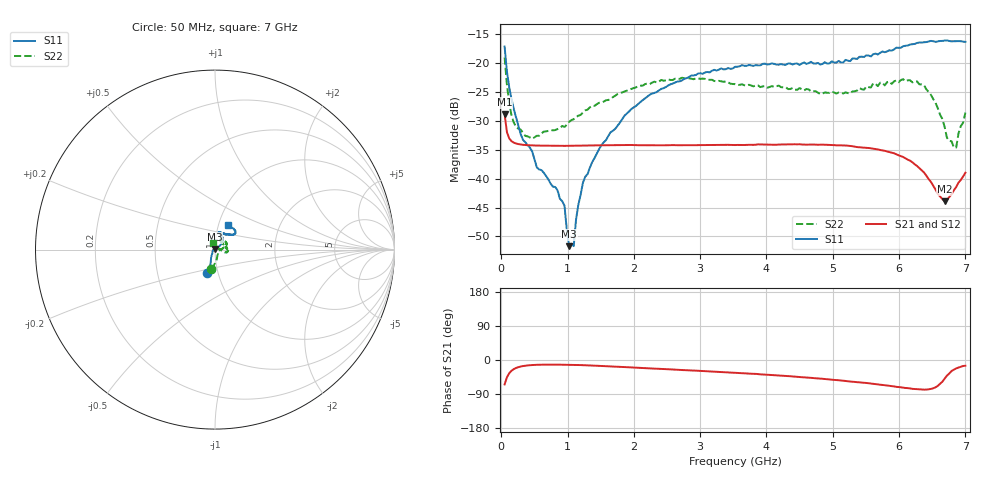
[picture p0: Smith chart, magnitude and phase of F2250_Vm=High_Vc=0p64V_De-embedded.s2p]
! Integrated Device Technology
! Corporate Headquarters
! 6024 Silver Creek Valley Road
! San Jose, CA 95138  USA
! Phone:  1-408-284-8200
! Toll Free:  1-800-223-1366
! Webpage:  http://www.idt.com/
! Timing and RF Division
! 515 Groton Road, Suite 102
! Westford, MA 01886-6024
! Device:  F2250
! Description: Voltage Variable RF Attenuator
! Frequency:  50.0 -  6000.00 MHz
! Package:  3x3 mm Thin QFN Plastic Package: 16 pin
! Ports:  2 RF, 3 DC
!  Pin  1  = GND
!  Pin  2  = NC
!  Pin  3  = RF1  = Port 1
!  Pin  4  = NC
!  Pin  5  = GND
!  Pin  6  = GND
!  Pin  7  = GND
!  Pin  8  = GND
!  Pin  9  = NC
!  Pin 10  = RF2  = Port 2
!  Pin 11  = NC
!  Pin 12  = GND
!  Pin 13  = GND
!  Pin 14  = VCNTRL
!  Pin 15  = VDD
!  Pin 16  = VMODE
! Vcntrl:  0.640 Volts
! Vmode:  +3.300 Volts
! Vdd:  +3.30  Volts
! Current:  1.281 mA
! Data:  The device was measured on a the F2250 evaluation board which has
!  individual transmission lines to the RF pins.  Data was collected
!  using a calibrated network analyzer.  The evaluation board was
!  de-embedded using a TRL calibration technique.
!  The reference plane is the edge of the package pin.
! Misc:  SN 10
!  Action Tracker AT0258
! Date Measured:  2014-11-26
! Date:  2015-10-15  MJV
! Note:
!  Integrated Device Technology supplies this data as a sample of measured
!  data at the package pin for this product.  Your particular data for this
!  product may vary.
!  Data was taken at 25 degrees C.
!  Integrated Device Technology reserves the right to change this data at anytime.
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# GHz S dB R 50
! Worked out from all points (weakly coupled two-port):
!   201 points, 50 MHz to 7 GHz, reference 50 ohm
!   highest |S21| = -28.86 dB at 50 MHz (marker M1); lowest = -43.9 dB at 6.687 GHz (marker M2)
!   lowest |S11| = -51.7 dB at 1.023 GHz (marker M3), VSWR 1.01, Z = 49.8 + j0.173 ohm
!   |S11| at or under -10 dB: start of sweep to end of sweep
!   |S22| runs from -34.6 to -19.1 dB; largest |S21 - S12| = 5.9e-05
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0.05  -17.17 -108.3  -28.86 -64.4  -28.86 -64.4  -19.06 -100.4
0.08475  -21.46 -107.1  -31.95 -45.7  -31.95 -45.7  -23.73 -83.9
0.1195  -24.21 -111.6  -33.04 -34.9  -33.04 -34.9  -26.96 -74.8
0.22375  -29.45 -121.9  -33.93 -20.9  -33.93 -21.0  -31.08 -52.1
0.5365  -38.07 -153.7  -34.28 -12.7  -34.28 -12.7  -32.59 -10.1
0.8145  -41.46 170.5  -34.33 -12.2  -34.33 -12.2  -31.60 0.1
0.9535  -44.68 171.6  -34.34 -12.5  -34.33 -12.5  -31.06 2.2
1.023  -51.68 138.1  -34.33 -12.7  -34.33 -12.7  -30.20 3.9
1.0925  -51.67 82.8  -34.32 -12.9  -34.31 -12.9  -29.72 5.4
1.12725  -47.10 57.1  -34.31 -13.1  -34.31 -13.1  -29.37 4.7
1.2315  -40.70 38.8  -34.28 -13.6  -34.28 -13.6  -28.55 4.1
1.6485  -31.98 40.4  -34.23 -16.8  -34.23 -16.8  -26.22 12.5
2.37825  -24.75 46.3  -34.22 -23.2  -34.22 -23.3  -23.21 22.9
3.525  -20.67 71.5  -34.20 -33.8  -34.20 -33.8  -23.67 50.9
4.7065  -20.08 71.9  -34.10 -47.7  -34.11 -47.7  -24.91 55.8
5.2625  -19.68 53.1  -34.35 -56.8  -34.34 -56.8  -25.29 31.3
5.85325  -17.80 40.4  -35.42 -68.1  -35.42 -68.2  -23.21 3.2
6.3745  -16.41 40.9  -38.92 -78.2  -38.94 -78.3  -23.79 -13.7
6.68725  -16.12 47.7  -43.95 -49.1  -43.94 -49.0  -31.08 4.3
6.722  -16.11 49.3  -43.65 -41.1  -43.62 -41.0  -32.94 10.5
6.861  -16.23 54.4  -41.45 -22.2  -41.43 -22.2  -34.62 62.9
7  -16.35 62.3  -38.98 -15.1  -38.94 -15.1  -28.60 103.7
